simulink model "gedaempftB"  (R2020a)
settings: Solver=ode45  StartTime=0.0  StopTime=10.0  RelTol=1e-3  EnableMultiTasking=on

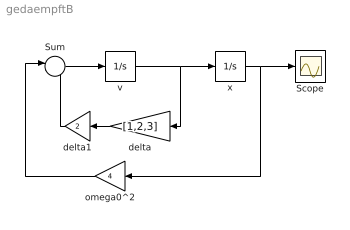
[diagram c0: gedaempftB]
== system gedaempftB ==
  Scope : Scope
  Sum : Sum  Inputs=|--  InputSameDT=on  SaturateOnIntegerOverflow=on
  delta : Gain  Gain=[1,2,3]  SaturateOnIntegerOverflow=on
  delta1 : Gain  Gain=2  SaturateOnIntegerOverflow=on
  omega0^2 : Gain  Gain=4  SaturateOnIntegerOverflow=on
  v : Integrator
  x : Integrator  InitialCondition=3
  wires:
  v/1 -> x/1, delta/1
  x/1 -> omega0^2/1, Scope/1
  Sum/1 -> v/1
  delta/1 -> delta1/1
  omega0^2/1 -> Sum/1
  delta1/1 -> Sum/2
